|Texas Instruments Incorporated
|IWRL6432AOP Single-Chip 60GHz mmWave Sensor
[IBIS Ver]   5.0
[Comment Char] |_char
[File name]   iwrl6432aop_fccsp101.ibs
[Date]   08/14/2025
[File Rev]   1.0
[Source]   Cadence Layout Workbench 22.1.4.12161.401368   004
[Notes]   Revision History:
| Rev 1.0: 08/14/2025
| - Initial version of the model
| - Note that QSPI[3] and OSC_CLK_OUT connect to 2 BGAs each, but only 1 of
|   each are listed in the header.
[Disclaimer]
| This model is designed as an aid for customers of Texas Instruments.
| TI and its licensors and suppliers make no warranties, either expressed
| or implied, with respect to this  model, including the warranties of
| merchantability or fitness for a particular purpose. The model is
| provided solely on an "as is" basis. The entire risk as to its quality
| and performance is with the customer.
| This model is subject to change without notice. Texas Instruments
| Incorporated is not responsible for updating this model.
[Copyright]
(C) Copyright 2022 Texas Instruments Incorporated.All rights reserved.
|  Component IWRL6432AOP_FCCSP 101-pin FCCSP - AMY0101 package
|  Part # IWRL6432AOP_FCCSP
[Component]   IWRL6432AOP_FCCSP
[Manufacturer]   Texas Instruments
[Package]   |101 FCCSP -AMY0101 package
|  variable   typ   min   max
R_pkg   0.14035   0.079117   0.32873
L_pkg   1.59e-9   9.678e-10   4.118e-9
C_pkg   3.763e-13   2.376e-13   8.832e-13
[Pin]   signal_name   model_name   R_pin   L_pin   C_pin
A1   VSS   GND   NA   NA   NA
A2   VPP   POWER   NA   NA   NA
A3   VSS   GND   NA   NA   NA
A4   VSS   GND   NA   NA   NA
A5   VSS   GND   NA   NA   NA
A6   VSSA   GND   NA   NA   NA
A7   VSSA   GND   NA   NA   NA
A8   OSC_CLK_OUT   NC   NA   NA   NA
A9   VSSA   GND   NA   NA   NA
A10   VSSA   GND   NA   NA   NA
B1   VIOIN_18   POWER   NA   NA   NA
B2   VPP   POWER   NA   NA   NA
B3   QSPI[3]   IO2   NA   NA   NA
B7   VSSA   GND   NA   NA   NA
B9   VSSA   GND   NA   NA   NA
B10   CLKM   NC   NA   NA   NA
C1   VIOIN   POWER   NA   NA   NA
C2   QSPI[0]   IO2   NA   NA   NA
C3   QSPI[1]   IO2   NA   NA   NA
C4   QSPI[2]   IO2   NA   NA   NA
C7   VDDA_10RF   POWER   NA   NA   NA
C8   VSSA   GND   NA   NA   NA
C9   VSSA   GND   NA   NA   NA
C10   VSSA   GND   NA   NA   NA
D2   QSPI_CLK   IO2   NA   NA   NA
D3   QSPI_CS   IO2   NA   NA   NA
D7   VIOIN_18CLK   POWER   NA   NA   NA
D8   VSSA   GND   NA   NA   NA
D9   VSSA   GND   NA   NA   NA
D10   CLKP   NC   NA   NA   NA
E1   VSS   GND   NA   NA   NA
E2   TDO   IO2   NA   NA   NA
E3   SPIA_MOSI   IO2   NA   NA   NA
E4   SPIA_MISO   IO2   NA   NA   NA
E7   VSSA   GND   NA   NA   NA
E8   VSSA   GND   NA   NA   NA
E9   VSSA   GND   NA   NA   NA
E10   VSSA   GND   NA   NA   NA
F1   SPIA_CLK   IO2   NA   NA   NA
F2   TDI   IO2   NA   NA   NA
F3   TCK   IO2   NA   NA   NA
F4   SPIA_CS0_N   IO2   NA   NA   NA
F7   VOUT_14SYNTH   NC   NA   NA   NA
F8   VSSA   GND   NA   NA   NA
F9   VDDA_18VCO   POWER   NA   NA   NA
F10   VDDA_18VCO   POWER   NA   NA   NA
G2   RS232_RX   IO2   NA   NA   NA
G3   TMS   IO2   NA   NA   NA
G8   VOUT_14APLL   NC   NA   NA   NA
G9   VSSA   GND   NA   NA   NA
G10   VSSA   GND   NA   NA   NA
H1   VSS   GND   NA   NA   NA
H2   GPIO_2   IO2   NA   NA   NA
H3   PMIC_CLKOUT   IO2   NA   NA   NA
H4   RS232_TX   IO2   NA   NA   NA
H7   VIN_18PM   POWER   NA   NA   NA
H8   VIN_18PM   POWER   NA   NA   NA
H9   VSSA   GND   NA   NA   NA
H10   VBGAP   NC   NA   NA   NA
J1   VIOIN   POWER   NA   NA   NA
J2   GPIO_5   IO1   NA   NA   NA
J3   UARTA_RX   IO1   NA   NA   NA
J4   NERROR_OUT   IO1   NA   NA   NA
J7   VSSA   GND   NA   NA   NA
J8   VSSA   GND   NA   NA   NA
J9   VSSA   GND   NA   NA   NA
J10   VSSA   GND   NA   NA   NA
K2   VDD   POWER   NA   NA   NA
K3   UARTA_TX   IO1   NA   NA   NA
K7   VDDA_10RF   POWER   NA   NA   NA
K8   VDDA_10RF   POWER   NA   NA   NA
K9   VDDA_10RF   POWER   NA   NA   NA
K10   VDDA_10RF   POWER   NA   NA   NA
L1   VIOIN_18   POWER   NA   NA   NA
L2   VIOIN_18   POWER   NA   NA   NA
L3   HOST_CLK_REQ   IO1   NA   NA   NA
L4   UARTA_RTS   IO1   NA   NA   NA
L7   VDDA_12RF   POWER   NA   NA   NA
L8   VDDA_12RF   POWER   NA   NA   NA
L9   VDDA_12RF   POWER   NA   NA   NA
L10   VDDA_12RF   POWER   NA   NA   NA
M1   VDD_SRAM   POWER   NA   NA   NA
M2   VNWA   POWER   NA   NA   NA
M3   NRESET   IOOD   NA   NA   NA
M7   VDDA_18BB   POWER   NA   NA   NA
M8   VDDA_18BB   POWER   NA   NA   NA
M9   VDDA_18BB   POWER   NA   NA   NA
M10   GPADC1   NC   NA   NA   NA
N1   VSS   GND   NA   NA   NA
N2   VNWA   POWER   NA   NA   NA
N3   VSS   GND   NA   NA   NA
N4   VSS   GND   NA   NA   NA
N5   VSS   GND   NA   NA   NA
N6   VDDA_18BB   POWER   NA   NA   NA
N7   VDDA_18BB   POWER   NA   NA   NA
N8   VDDA_18BB   POWER   NA   NA   NA
N9   VDDA_18BB   POWER   NA   NA   NA
N10   VDDA_18BB   POWER   NA   NA   NA
| Model IOOD
[Model Selector] IOOD
|SC1 IS A SLEW RATE CONTROL PIN
|5% SUPPLY VARIATION MODES WITH 1.8V NOM SUPPLY
IOOD_V_PUPDOFF_5P_SC1_1P8  Cell operated at 1.8(nom)
|IOOD_V_PUPDOFF_5P_SC1_1P8; BUFFER WITH WEAK PULUP/PULLDOWN OFF AT 5% SUPPLY
|VARIATION WITH SC1=1 MEANING SLOW MODE OF OPERATION
IOOD_V_PD_ON_5P_!SC1_1P8  Cell operated at 1.8(nom)
|IOOD_V_PD_ON_5P_!SC1_1P8; BUFFER WITH WEAK_PULLDOWN_ON AT 5% SUPPLY
|VARIATION WITH SC1=0 MEANING FAST MODE OF OPERATION
IOOD_V_PD_ON_5P_SC1_1P8  Cell operated at 1.8(nom)
|IOOD_V_PD_ON_5P_SC1_1P8; BUFFER WITH WEAK_PULLDOWN_ON AT 5% SUPPLY
|VARIATION WITH SC1=1 MEANING SLOW MODE OF OPERATION
IOOD_V_PU_ON_5P_!SC1_1P8  Cell operated at 1.8(nom)
|IOOD_V_PU_ON_5P_!SC1_1P8; BUFFER WITH WEAK_PULLUP_ON AT 5% SUPPLY
|VARIATION WITH SC1=0 MEANING FAST MODE OF OPERATION
IOOD_V_PUPDOFF_5P_!SC1_1P8  Cell operated at 1.8(nom)
|IOOD_V_PUPDOFF_5P_!SC1_1P8; BUFFER WITH WEAK PULUP/PULLDOWN OFF AT 5% SUPPLY
|VARIATION WITH SC1=0 MEANING FAST MODE OF OPERATION
IOOD_V_PU_ON_5P_SC1_1P8  Cell operated at 1.8(nom)
|IOOD_V_PU_ON_5P_SC1_1P8; BUFFER WITH WEAK_PULLUP_ON AT 5% SUPPLY
|VARIATION WITH SC1=1 MEANING SLOW MODE OF OPERATION
|5% SUPPLY VARIATION MODES WITH 3.3V NOM SUPPLY
IOOD_V_PUPDOFF_5P_SC1_3P3  Cell operated at 3.3(nom)
|IOOD_V_PUPDOFF_5P_SC1_3P3; BUFFER WITH WEAK PULUP/PULLDOWN OFF AT 5% SUPPLY
|VARIATION WITH SC1=1 MEANING SLOW MODE OF OPERATION
IOOD_V_PD_ON_5P_!SC1_3P3  Cell operated at 3.3(nom)
|IOOD_V_PD_ON_5P_!SC1_3P3; BUFFER WITH WEAK_PULLDOWN_ON AT 5% SUPPLY
|VARIATION WITH SC1=0 MEANING FAST MODE OF OPERATION
IOOD_V_PD_ON_5P_SC1_3P3  Cell operated at 3.3(nom)
|IOOD_V_PD_ON_5P_SC1_3P3; BUFFER WITH WEAK_PULLDOWN_ON AT 5% SUPPLY
|VARIATION WITH SC1=1 MEANING SLOW MODE OF OPERATION
IOOD_V_PU_ON_5P_!SC1_3P3  Cell operated at 3.3(nom)
|IOOD_V_PU_ON_5P_!SC1_3P3; BUFFER WITH WEAK_PULLUP_ON AT 5% SUPPLY
|VARIATION WITH SC1=0 MEANING FAST MODE OF OPERATION
IOOD_V_PUPDOFF_5P_!SC1_3P3  Cell operated at 3.3(nom)
|IOOD_V_PUPDOFF_5P_!SC1_3P3; BUFFER WITH WEAK PULUP/PULLDOWN OFF AT 5% SUPPLY
|VARIATION WITH SC1=0 MEANING FAST MODE OF OPERATION
IOOD_V_PU_ON_5P_SC1_3P3  Cell operated at 3.3(nom)
|IOOD_V_PU_ON_5P_SC1_3P3; BUFFER WITH WEAK_PULLUP_ON AT 5% SUPPLY
|VARIATION WITH SC1=1 MEANING SLOW MODE OF OPERATION
| 10% SUPPLY VARIATION MODES WITH 1.8V NOM SUPPLY
IOOD_V_PUPDOFF_10P_SC1_1P8  Cell operated at 1.8(nom)
|IOOD_V_PUPDOFF_10P_SC1_1P8; BUFFER WITH WEAK PULUP/PULLDOWN OFF AT 10% SUPPLY
|VARIATION WITH SC1=1 MEANING SLOW MODE OF OPERATION
IOOD_V_PD_ON_10P_!SC1_1P8  Cell operated at 1.8(nom)
|IOOD_V_PD_ON_10P_!SC1_1P8; BUFFER WITH WEAK_PULLDOWN_ON AT 10% SUPPLY
|VARIATION WITH SC1=0 MEANING FAST MODE OF OPERATION
IOOD_V_PD_ON_10P_SC1_1P8  Cell operated at 1.8(nom)
|IOOD_V_PD_ON_10P_SC1_1P8; BUFFER WITH WEAK_PULLDOWN_ON AT 10% SUPPLY
|VARIATION WITH SC1=1 MEANING SLOW MODE OF OPERATION
IOOD_V_PU_ON_10P_!SC1_1P8  Cell operated at 1.8(nom)
|IOOD_V_PU_ON_10P_!SC1_1P8; BUFFER WITH WEAK_PULLUP_ON AT 10% SUPPLY
|VARIATION WITH SC1=0 MEANING FAST MODE OF OPERATION
IOOD_V_PUPDOFF_10P_!SC1_1P8  Cell operated at 1.8(nom)
|IOOD_V_PUPDOFF_10P_!SC1_1P8; BUFFER WITH WEAK PULUP/PULLDOWN OFF AT 10% SUPPLY
|VARIATION WITH SC1=0 MEANING FAST MODE OF OPERATION
IOOD_V_PU_ON_10P_SC1_1P8  Cell operated at 1.8(nom)
|IOOD_V_PU_ON_10P_SC1_1P8; BUFFER WITH WEAK_PULLUP_ON AT 10% SUPPLY
|VARIATION WITH SC1=1 MEANING SLOW MODE OF OPERATION
| 10% SUPPLY VARIATION MODES WITH 3.3V NOM SUPPLY
IOOD_V_PUPDOFF_10P_SC1_3P3  Cell operated at 3.3(nom)
|IOOD_V_PUPDOFF_10P_SC1_3P3; BUFFER WITH WEAK PULUP/PULLDOWN OFF AT 10% SUPPLY
|VARIATION WITH SC1=1 MEANING SLOW MODE OF OPERATION
IOOD_V_PD_ON_10P_!SC1_3P3  Cell operated at 3.3(nom)
|IOOD_V_PD_ON_10P_!SC1_3P3; BUFFER WITH WEAK_PULLDOWN_ON 10% SUPPLY
|VARIATION WITH SC1=0 MEANING FAST MODE OF OPERATION
IOOD_V_PD_ON_10P_SC1_3P3  Cell operated at 3.3(nom)
|IOOD_V_PD_ON_10P_SC1_3P3; BUFFER WITH WEAK_PULLDOWN_ON AT 10% SUPPLY
|VARIATION WITH SC1=1 MEANING SLOW MODE OF OPERATION
IOOD_V_PU_ON_10P_!SC1_3P3  Cell operated at 3.3(nom)
|IOOD_V_PU_ON_10P_!SC1_3P3; BUFFER WITH WEAK_PULLUP_ON AT 10% SUPPLY
|VARIATION WITH SC1=0 MEANING FAST MODE OF OPERATION
IOOD_V_PUPDOFF_10P_!SC1_3P3  Cell operated at 3.3(nom)
|IOOD_V_PUPDOFF_10P_!SC1_3P3; BUFFER WITH WEAK PULUP/PULLDOWN OFF AT 10% SUPPLY
|VARIATION WITH SC1=0 MEANING FAST MODE OF OPERATION
IOOD_V_PU_ON_10P_SC1_3P3  Cell operated at 3.3(nom)
|IOOD_V_PU_ON_10P_SC1_3P3; BUFFER WITH WEAK_PULLUP_ON AT 10% SUPPLY
|VARIATION WITH SC1=1 MEANING SLOW MODE OF OPERATION
| Model IO1
[Model Selector] IO1
|SC1 IS A SLEW RATE CONTROL PIN
|5% SUPPLY VARIATION MODES WITH 1.8V NOM SUPPLY
BC40D_V_PUPDOFF_5P_SC1_1P8  Cell operated at 1.8(nom)
|BC40D_V_PUPDOFF_5P_SC1_1P8; BUFFER WITH WEAK PULUP/PULLDOWN OFF AT 5% SUPPLY
|VARIATION WITH SC1=1 MEANING SLOW MODE OF OPERATION
BC40D_V_PD_ON_5P_!SC1_1P8  Cell operated at 1.8(nom)
|BC40D_V_PD_ON_5P_!SC1_1P8; BUFFER WITH WEAK_PULLDOWN_ON AT 5% SUPPLY
|VARIATION WITH SC1=0 MEANING FAST MODE OF OPERATION
BC40D_V_PD_ON_5P_SC1_1P8  Cell operated at 1.8(nom)
|BC40D_V_PD_ON_5P_SC1_1P8; BUFFER WITH WEAK_PULLDOWN_ON AT 5% SUPPLY
|VARIATION WITH SC1=1 MEANING SLOW MODE OF OPERATION
BC40D_V_PU_ON_5P_!SC1_1P8  Cell operated at 1.8(nom)
|BC40D_V_PU_ON_5P_!SC1_1P8; BUFFER WITH WEAK_PULLUP_ON AT 5% SUPPLY
|VARIATION WITH SC1=0 MEANING FAST MODE OF OPERATION
BC40D_V_PUPDOFF_5P_!SC1_1P8  Cell operated at 1.8(nom)
|BC40D_V_PUPDOFF_5P_!SC1_1P8; BUFFER WITH WEAK PULUP/PULLDOWN OFF AT 5% SUPPLY
|VARIATION WITH SC1=0 MEANING FAST MODE OF OPERATION
BC40D_V_PU_ON_5P_SC1_1P8  Cell operated at 1.8(nom)
|BC40D_V_PU_ON_5P_SC1_1P8; BUFFER WITH WEAK_PULLUP_ON AT 5% SUPPLY
|VARIATION WITH SC1=1 MEANING SLOW MODE OF OPERATION
|5% SUPPLY VARIATION MODES WITH 3.3V NOM SUPPLY
BC40D_V_PUPDOFF_5P_SC1_3P3  Cell operated at 3.3(nom)
|BC40D_V_PUPDOFF_5P_SC1_3P3; BUFFER WITH WEAK PULUP/PULLDOWN OFF AT 5% SUPPLY
|VARIATION WITH SC1=1 MEANING SLOW MODE OF OPERATION
BC40D_V_PD_ON_5P_!SC1_3P3  Cell operated at 3.3(nom)
|BC40D_V_PD_ON_5P_!SC1_3P3; BUFFER WITH WEAK_PULLDOWN_ON AT 5% SUPPLY
|VARIATION WITH SC1=0 MEANING FAST MODE OF OPERATION
BC40D_V_PD_ON_5P_SC1_3P3  Cell operated at 3.3(nom)
|BC40D_V_PD_ON_5P_SC1_3P3; BUFFER WITH WEAK_PULLDOWN_ON AT 5% SUPPLY
|VARIATION WITH SC1=1 MEANING SLOW MODE OF OPERATION
BC40D_V_PU_ON_5P_!SC1_3P3  Cell operated at 3.3(nom)
|BC40D_V_PU_ON_5P_!SC1_3P3; BUFFER WITH WEAK_PULLUP_ON AT 5% SUPPLY
|VARIATION WITH SC1=0 MEANING FAST MODE OF OPERATION
BC40D_V_PUPDOFF_5P_!SC1_3P3  Cell operated at 3.3(nom)
|BC40D_V_PUPDOFF_5P_!SC1_3P3; BUFFER WITH WEAK PULUP/PULLDOWN OFF AT 5% SUPPLY
|VARIATION WITH SC1=0 MEANING FAST MODE OF OPERATION
BC40D_V_PU_ON_5P_SC1_3P3  Cell operated at 3.3(nom)
|BC40D_V_PU_ON_5P_SC1_3P3; BUFFER WITH WEAK_PULLUP_ON AT 5% SUPPLY
|VARIATION WITH SC1=1 MEANING SLOW MODE OF OPERATION
| 10% SUPPLY VARIATION MODES WITH 1.8V NOM SUPPLY
BC40D_V_PUPDOFF_10P_SC1_1P8  Cell operated at 1.8(nom)
|BC40D_V_PUPDOFF_10P_SC1_1P8; BUFFER WITH WEAK PULUP/PULLDOWN OFF AT 10% SUPPLY
|VARIATION WITH SC1=1 MEANING SLOW MODE OF OPERATION
BC40D_V_PD_ON_10P_!SC1_1P8  Cell operated at 1.8(nom)
|BC40D_V_PD_ON_10P_!SC1_1P8; BUFFER WITH WEAK_PULLDOWN_ON AT 10% SUPPLY
|VARIATION WITH SC1=0 MEANING FAST MODE OF OPERATION
BC40D_V_PD_ON_10P_SC1_1P8  Cell operated at 1.8(nom)
|BC40D_V_PD_ON_10P_SC1_1P8; BUFFER WITH WEAK_PULLDOWN_ON AT 10% SUPPLY
|VARIATION WITH SC1=1 MEANING SLOW MODE OF OPERATION
BC40D_V_PU_ON_10P_!SC1_1P8  Cell operated at 1.8(nom)
|BC40D_V_PU_ON_10P_!SC1_1P8; BUFFER WITH WEAK_PULLUP_ON AT 10% SUPPLY
|VARIATION WITH SC1=0 MEANING FAST MODE OF OPERATION
BC40D_V_PUPDOFF_10P_!SC1_1P8  Cell operated at 1.8(nom)
|BC40D_V_PUPDOFF_10P_!SC1_1P8; BUFFER WITH WEAK PULUP/PULLDOWN OFF AT 10% SUPPLY
|VARIATION WITH SC1=0 MEANING FAST MODE OF OPERATION
BC40D_V_PU_ON_10P_SC1_1P8  Cell operated at 1.8(nom)
|BC40D_V_PU_ON_10P_SC1_1P8; BUFFER WITH WEAK_PULLUP_ON AT 10% SUPPLY
|VARIATION WITH SC1=1 MEANING SLOW MODE OF OPERATION
| 10% SUPPLY VARIATION MODES WITH 3.3V NOM SUPPLY
BC40D_V_PUPDOFF_10P_SC1_3P3  Cell operated at 3.3(nom)
|BC40D_V_PUPDOFF_10P_SC1_3P3; BUFFER WITH WEAK PULUP/PULLDOWN OFF AT 10% SUPPLY
|VARIATION WITH SC1=1 MEANING SLOW MODE OF OPERATION
BC40D_V_PD_ON_10P_!SC1_3P3  Cell operated at 3.3(nom)
|BC40D_V_PD_ON_10P_!SC1_3P3; BUFFER WITH WEAK_PULLDOWN_ON 10% SUPPLY
|VARIATION WITH SC1=0 MEANING FAST MODE OF OPERATION
BC40D_V_PD_ON_10P_SC1_3P3  Cell operated at 3.3(nom)
|BC40D_V_PD_ON_10P_SC1_3P3; BUFFER WITH WEAK_PULLDOWN_ON AT 10% SUPPLY
|VARIATION WITH SC1=1 MEANING SLOW MODE OF OPERATION
BC40D_V_PU_ON_10P_!SC1_3P3  Cell operated at 3.3(nom)
|BC40D_V_PU_ON_10P_!SC1_3P3; BUFFER WITH WEAK_PULLUP_ON AT 10% SUPPLY
|VARIATION WITH SC1=0 MEANING FAST MODE OF OPERATION
BC40D_V_PUPDOFF_10P_!SC1_3P3  Cell operated at 3.3(nom)
|BC40D_V_PUPDOFF_10P_!SC1_3P3; BUFFER WITH WEAK PULUP/PULLDOWN OFF AT 10% SUPPLY
|VARIATION WITH SC1=0 MEANING FAST MODE OF OPERATION
BC40D_V_PU_ON_10P_SC1_3P3  Cell operated at 3.3(nom)
|BC40D_V_PU_ON_10P_SC1_3P3; BUFFER WITH WEAK_PULLUP_ON AT 10% SUPPLY
|VARIATION WITH SC1=1 MEANING SLOW MODE OF OPERATION
| Model IO2
[Model Selector] IO2
|SC1 IS A SLEW RATE CONTROL PIN
|5% SUPPLY VARIATION MODES WITH 1.8V NOM SUPPLY
BC40D_H_PUPDOFF_5P_SC1_1P8  Cell operated at 1.8(nom)
|BC40D_H_PUPDOFF_5P_SC1_1P8; BUFFER WITH WEAK PULUP/PULLDOWN OFF AT 5% SUPPLY
|VARIATION WITH SC1=1 MEANING SLOW MODE OF OPERATION
BC40D_H_PD_ON_5P_!SC1_1P8  Cell operated at 1.8(nom)
|BC40D_H_PD_ON_5P_!SC1_1P8; BUFFER WITH WEAK_PULLDOWN_ON AT 5% SUPPLY
|VARIATION WITH SC1=0 MEANING FAST MODE OF OPERATION
BC40D_H_PD_ON_5P_SC1_1P8  Cell operated at 1.8(nom)
|BC40D_H_PD_ON_5P_SC1_1P8; BUFFER WITH WEAK_PULLDOWN_ON AT 5% SUPPLY
|VARIATION WITH SC1=1 MEANING SLOW MODE OF OPERATION
BC40D_H_PU_ON_5P_!SC1_1P8  Cell operated at 1.8(nom)
|BC40D_H_PU_ON_5P_!SC1_1P8; BUFFER WITH WEAK_PULLUP_ON AT 5% SUPPLY
|VARIATION WITH SC1=0 MEANING FAST MODE OF OPERATION
BC40D_H_PUPDOFF_5P_!SC1_1P8  Cell operated at 1.8(nom)
|BC40D_H_PUPDOFF_5P_!SC1_1P8; BUFFER WITH WEAK PULUP/PULLDOWN OFF AT 5% SUPPLY
|VARIATION WITH SC1=0 MEANING FAST MODE OF OPERATION
BC40D_H_PU_ON_5P_SC1_1P8  Cell operated at 1.8(nom)
|BC40D_H_PU_ON_5P_SC1_1P8; BUFFER WITH WEAK_PULLUP_ON AT 5% SUPPLY
|VARIATION WITH SC1=1 MEANING SLOW MODE OF OPERATION
|5% SUPPLY VARIATION MODES WITH 3.3V NOM SUPPLY
BC40D_H_PUPDOFF_5P_SC1_3P3  Cell operated at 3.3(nom)
|BC40D_H_PUPDOFF_5P_SC1_3P3; BUFFER WITH WEAK PULUP/PULLDOWN OFF AT 5% SUPPLY
|VARIATION WITH SC1=1 MEANING SLOW MODE OF OPERATION
BC40D_H_PD_ON_5P_!SC1_3P3  Cell operated at 3.3(nom)
|BC40D_H_PD_ON_5P_!SC1_3P3; BUFFER WITH WEAK_PULLDOWN_ON AT 5% SUPPLY
|VARIATION WITH SC1=0 MEANING FAST MODE OF OPERATION
BC40D_H_PD_ON_5P_SC1_3P3  Cell operated at 3.3(nom)
|BC40D_H_PD_ON_5P_SC1_3P3; BUFFER WITH WEAK_PULLDOWN_ON AT 5% SUPPLY
|VARIATION WITH SC1=1 MEANING SLOW MODE OF OPERATION
BC40D_H_PU_ON_5P_!SC1_3P3  Cell operated at 3.3(nom)
|BC40D_H_PU_ON_5P_!SC1_3P3; BUFFER WITH WEAK_PULLUP_ON AT 5% SUPPLY
|VARIATION WITH SC1=0 MEANING FAST MODE OF OPERATION
BC40D_H_PUPDOFF_5P_!SC1_3P3  Cell operated at 3.3(nom)
|BC40D_H_PUPDOFF_5P_!SC1_3P3; BUFFER WITH WEAK PULUP/PULLDOWN OFF AT 5% SUPPLY
|VARIATION WITH SC1=0 MEANING FAST MODE OF OPERATION
BC40D_H_PU_ON_5P_SC1_3P3  Cell operated at 3.3(nom)
|BC40D_H_PU_ON_5P_SC1_3P3; BUFFER WITH WEAK_PULLUP_ON AT 5% SUPPLY
|VARIATION WITH SC1=1 MEANING SLOW MODE OF OPERATION
| 10% SUPPLY VARIATION MODES WITH 1.8V NOM SUPPLY
BC40D_H_PUPDOFF_10P_SC1_1P8  Cell operated at 1.8(nom)
|BC40D_H_PUPDOFF_10P_SC1_1P8; BUFFER WITH WEAK PULUP/PULLDOWN OFF AT 10% SUPPLY
|VARIATION WITH SC1=1 MEANING SLOW MODE OF OPERATION
BC40D_H_PD_ON_10P_!SC1_1P8  Cell operated at 1.8(nom)
|BC40D_H_PD_ON_10P_!SC1_1P8; BUFFER WITH WEAK_PULLDOWN_ON AT 10% SUPPLY
|VARIATION WITH SC1=0 MEANING FAST MODE OF OPERATION
BC40D_H_PD_ON_10P_SC1_1P8  Cell operated at 1.8(nom)
|BC40D_H_PD_ON_10P_SC1_1P8; BUFFER WITH WEAK_PULLDOWN_ON AT 10% SUPPLY
|VARIATION WITH SC1=1 MEANING SLOW MODE OF OPERATION
BC40D_H_PU_ON_10P_!SC1_1P8  Cell operated at 1.8(nom)
|BC40D_H_PU_ON_10P_!SC1_1P8; BUFFER WITH WEAK_PULLUP_ON AT 10% SUPPLY
|VARIATION WITH SC1=0 MEANING FAST MODE OF OPERATION
BC40D_H_PUPDOFF_10P_!SC1_1P8  Cell operated at 1.8(nom)
|BC40D_H_PUPDOFF_10P_!SC1_1P8; BUFFER WITH WEAK PULUP/PULLDOWN OFF AT 10% SUPPLY
|VARIATION WITH SC1=0 MEANING FAST MODE OF OPERATION
BC40D_H_PU_ON_10P_SC1_1P8  Cell operated at 1.8(nom)
|BC40D_H_PU_ON_10P_SC1_1P8; BUFFER WITH WEAK_PULLUP_ON AT 10% SUPPLY
|VARIATION WITH SC1=1 MEANING SLOW MODE OF OPERATION
| 10% SUPPLY VARIATION MODES WITH 3.3V NOM SUPPLY
BC40D_H_PUPDOFF_10P_SC1_3P3  Cell operated at 3.3(nom)
|BC40D_H_PUPDOFF_10P_SC1_3P3; BUFFER WITH WEAK PULUP/PULLDOWN OFF AT 10% SUPPLY
|VARIATION WITH SC1=1 MEANING SLOW MODE OF OPERATION
BC40D_H_PD_ON_10P_!SC1_3P3  Cell operated at 3.3(nom)
|BC40D_H_PD_ON_10P_!SC1_3P3; BUFFER WITH WEAK_PULLDOWN_ON 10% SUPPLY
|VARIATION WITH SC1=0 MEANING FAST MODE OF OPERATION
BC40D_H_PD_ON_10P_SC1_3P3  Cell operated at 3.3(nom)
|BC40D_H_PD_ON_10P_SC1_3P3; BUFFER WITH WEAK_PULLDOWN_ON AT 10% SUPPLY
|VARIATION WITH SC1=1 MEANING SLOW MODE OF OPERATION
BC40D_H_PU_ON_10P_!SC1_3P3  Cell operated at 3.3(nom)
|BC40D_H_PU_ON_10P_!SC1_3P3; BUFFER WITH WEAK_PULLUP_ON AT 10% SUPPLY
|VARIATION WITH SC1=0 MEANING FAST MODE OF OPERATION
BC40D_H_PUPDOFF_10P_!SC1_3P3  Cell operated at 3.3(nom)
|BC40D_H_PUPDOFF_10P_!SC1_3P3; BUFFER WITH WEAK PULUP/PULLDOWN OFF AT 10% SUPPLY
|VARIATION WITH SC1=0 MEANING FAST MODE OF OPERATION
BC40D_H_PU_ON_10P_SC1_3P3  Cell operated at 3.3(nom)
[Define Package Model]   IWRL6432AOP_FCCSP
[Manufacturer]   TI
[OEM]   TI
[Description]   FCCSP
|[Number of Sections]   1
[Number of Pins]   44
[Pin Numbers]
|[Pin Name]  Net Number   Net Name   Net's All Pins
H10   | 1   VBGAP   H10
K2   | 2   VDD   K2
K10   | 3   VDDA_10RF   K10
   |K9
   |K8
   |K7
   |C7
L10   | 4   VDDA_12RF   L10
   |L9
   |L8
   |L7
N10   | 5   VDDA_18BB   N10
   |M9
   |N9
   |M8
   |M7
   |N8
   |N7
F10   | 6   VDDA_18VCO   F10
   |F9
M1   | 7   VDD_SRAM   M1
H8   | 8   VIN_18PM   H8
   |H7
J1   | 9   VIOIN   J1
   |C1
L2   | 10   VIOIN_18   L2
   |L1
   |B1
D7   | 11   VIOIN_18CLK   D7
N2   | 12   VNWA   N2
   |M2
G8   | 13   VOUT_14APLL   G8
F7   | 14   VOUT_14SYNTH   F7
A2   | 15   VPP   A2
   |B2
B10   | 16   CLKM   B10
D10   | 17   CLKP   D10
M10   | 18   GPADC1   M10
H2   | 19   GPIO_2   H2
J2   | 20   GPIO_5   J2
L3   | 21   HOST_CLK_REQ   L3
J4   | 22   NERROR_OUT   J4
M3   | 23   NRESET   M3
   |M4
A8   | 24   OSC_CLK_OUT   A8
   |B8
H3   | 25   PMIC_CLKOUT   H3
C2   | 26   QSPI[0]   C2
C3   | 27   QSPI[1]   C3
C4   | 28   QSPI[2]   C4
B3   | 29   QSPI[3]   B3
   |B4
D2   | 30   QSPI_CLK   D2
D3   | 31   QSPI_CS   D3
G2   | 32   RS232_RX   G2
H4   | 33   RS232_TX   H4
F1   | 34   SPIA_CLK   F1
F4   | 35   SPIA_CS0_N   F4
E4   | 36   SPIA_MISO   E4
E3   | 37   SPIA_MOSI   E3
F3   | 38   TCK   F3
F2   | 39   TDI   F2
E2   | 40   TDO   E2
G3   | 41   TMS   G3
L4   | 42   UARTA_RTS   L4
J3   | 43   UARTA_RX   J3
K3   | 44   UARTA_TX   K3
[Model Data]
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[End Model Data]
[End Package Model]
| Models and submodels in the file (72): BC40D_V_PUPDOFF_5P_SC1_1P8 (I/O), BC40D_V_PD_ON_5P_!SC1_1P8 (I/O), BC40D_V_PD_ON_5P_SC1_1P8 (I/O), BC40D_V_PU_ON_5P_!SC1_1P8 (I/O), BC40D_V_PUPDOFF_5P_!SC1_1P8 (I/O), BC40D_V_PU_ON_5P_SC1_1P8 (I/O), BC40D_V_PUPDOFF_5P_SC1_3P3 (I/O), BC40D_V_PD_ON_5P_!SC1_3P3 (I/O), BC40D_V_PD_ON_5P_SC1_3P3 (I/O), BC40D_V_PU_ON_5P_!SC1_3P3 (I/O), BC40D_V_PUPDOFF_5P_!SC1_3P3 (I/O), BC40D_V_PU_ON_5P_SC1_3P3 (I/O), BC40D_V_PUPDOFF_10P_SC1_1P8 (I/O), BC40D_V_PD_ON_10P_!SC1_1P8 (I/O), BC40D_V_PD_ON_10P_SC1_1P8 (I/O), BC40D_V_PU_ON_10P_!SC1_1P8 (I/O), BC40D_V_PUPDOFF_10P_!SC1_1P8 (I/O), BC40D_V_PU_ON_10P_SC1_1P8 (I/O), BC40D_V_PUPDOFF_10P_SC1_3P3 (I/O), BC40D_V_PD_ON_10P_!SC1_3P3 (I/O), BC40D_V_PD_ON_10P_SC1_3P3 (I/O), BC40D_V_PU_ON_10P_!SC1_3P3 (I/O), BC40D_V_PUPDOFF_10P_!SC1_3P3 (I/O), BC40D_V_PU_ON_10P_SC1_3P3 (I/O), BC40D_H_PUPDOFF_5P_SC1_1P8 (I/O), BC40D_H_PD_ON_5P_!SC1_1P8 (I/O), BC40D_H_PD_ON_5P_SC1_1P8 (I/O), BC40D_H_PU_ON_5P_!SC1_1P8 (I/O), BC40D_H_PUPDOFF_5P_!SC1_1P8 (I/O), BC40D_H_PU_ON_5P_SC1_1P8 (I/O), BC40D_H_PUPDOFF_5P_SC1_3P3 (I/O), BC40D_H_PD_ON_5P_!SC1_3P3 (I/O), BC40D_H_PD_ON_5P_SC1_3P3 (I/O), BC40D_H_PU_ON_5P_!SC1_3P3 (I/O), BC40D_H_PUPDOFF_5P_!SC1_3P3 (I/O), BC40D_H_PU_ON_5P_SC1_3P3 (I/O), BC40D_H_PUPDOFF_10P_SC1_1P8 (I/O), BC40D_H_PD_ON_10P_!SC1_1P8 (I/O), BC40D_H_PD_ON_10P_SC1_1P8 (I/O), BC40D_H_PU_ON_10P_!SC1_1P8 (I/O), BC40D_H_PUPDOFF_10P_!SC1_1P8 (I/O), BC40D_H_PU_ON_10P_SC1_1P8 (I/O), BC40D_H_PUPDOFF_10P_SC1_3P3 (I/O), BC40D_H_PD_ON_10P_!SC1_3P3 (I/O), BC40D_H_PD_ON_10P_SC1_3P3 (I/O), BC40D_H_PU_ON_10P_!SC1_3P3 (I/O), BC40D_H_PUPDOFF_10P_!SC1_3P3 (I/O), BC40D_H_PU_ON_10P_SC1_3P3 (I/O), IOOD_V_PUPDOFF_5P_SC1_1P8 (I/O_open_drain), IOOD_V_PD_ON_5P_!SC1_1P8 (I/O_open_drain), IOOD_V_PD_ON_5P_SC1_1P8 (I/O_open_drain), IOOD_V_PU_ON_5P_!SC1_1P8 (I/O_open_drain), IOOD_V_PUPDOFF_5P_!SC1_1P8 (I/O_open_drain), IOOD_V_PU_ON_5P_SC1_1P8 (I/O_open_drain), IOOD_V_PUPDOFF_5P_SC1_3P3 (I/O_open_drain), IOOD_V_PD_ON_5P_!SC1_3P3 (I/O_open_drain), IOOD_V_PD_ON_5P_SC1_3P3 (I/O_open_drain), IOOD_V_PU_ON_5P_!SC1_3P3 (I/O_open_drain), IOOD_V_PUPDOFF_5P_!SC1_3P3 (I/O_open_drain), IOOD_V_PU_ON_5P_SC1_3P3 (I/O_open_drain), IOOD_V_PUPDOFF_10P_SC1_1P8 (I/O_open_drain), IOOD_V_PD_ON_10P_!SC1_1P8 (I/O_open_drain), IOOD_V_PD_ON_10P_SC1_1P8 (I/O_open_drain), IOOD_V_PU_ON_10P_!SC1_1P8 (I/O_open_drain), IOOD_V_PUPDOFF_10P_!SC1_1P8 (I/O_open_drain), IOOD_V_PU_ON_10P_SC1_1P8 (I/O_open_drain), IOOD_V_PUPDOFF_10P_SC1_3P3 (I/O_open_drain), IOOD_V_PD_ON_10P_!SC1_3P3 (I/O_open_drain), IOOD_V_PD_ON_10P_SC1_3P3 (I/O_open_drain), IOOD_V_PU_ON_10P_!SC1_3P3 (I/O_open_drain), IOOD_V_PUPDOFF_10P_!SC1_3P3 (I/O_open_drain), IOOD_V_PU_ON_10P_SC1_3P3 (I/O_open_drain)
